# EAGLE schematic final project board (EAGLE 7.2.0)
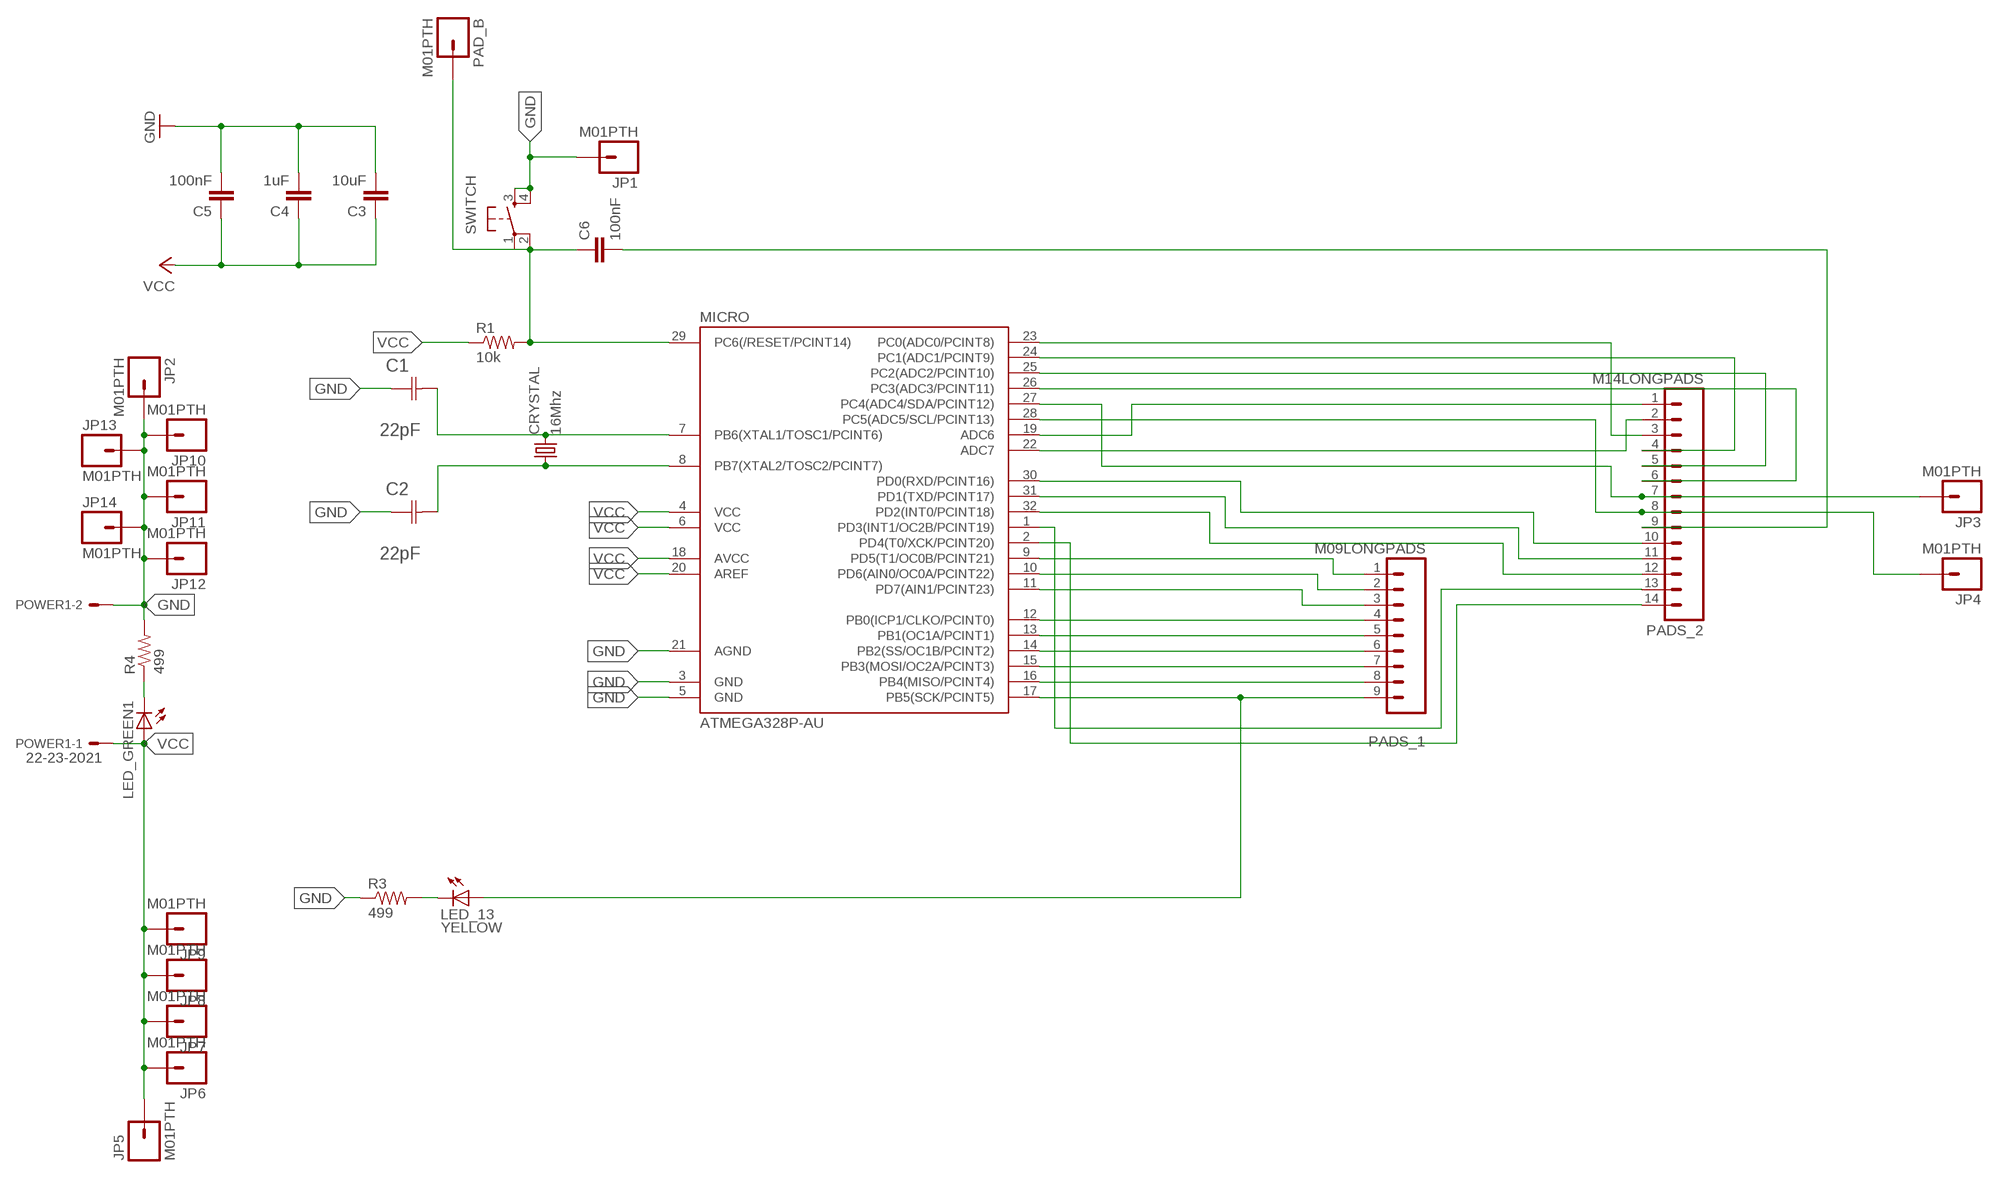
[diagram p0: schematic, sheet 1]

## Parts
C1  22pF  0612ZC225MAT2A  [CAPC3216X178N]
C2  22pF  0612ZC225MAT2A  [CAPC3216X178N]
C3  10uF  CAP1206  [1206]
C4  1uF  CAP1206  [1206]
C5  100nF  CAP1206  [1206]
C6  100nF  CAP1206  [1206]
CRYSTAL  16Mhz  CSM-7X-DU  [CSM-7X-DU]
JP1  M01PTH  [1X01]
JP2  M01PTH  [1X01]
JP3  M01PTH  [1X01]
JP4  M01PTH  [1X01]
JP5  M01PTH  [1X01]
JP6  M01PTH  [1X01]
JP7  M01PTH  [1X01]
JP8  M01PTH  [1X01]
JP9  M01PTH  [1X01]
JP10  M01PTH  [1X01]
JP11  M01PTH  [1X01]
JP12  M01PTH  [1X01]
JP13  M01PTH  [1X01]
JP14  M01PTH  [1X01]
LED_13  YELLOW  LED1206  [1206]
LED_GREEN1  LED1206  [1206]
MICRO  ATMEGA328P-AU  ATMEGA48/88/168-AU  [TQFP32-08]
PAD_B  M01PTH  [1X01]
PADS_1  M09LONGPADS  [1X09_LONGPADS]
PADS_2  M14LONGPADS  [1X14-LONGPADS]
POWER1  22-23-2021  [22-23-2021]
R1  10k  RESISTOR1206  [1206]
R3  499  RESISTOR1206  [1206]
R4  499  RESISTOR1206  [1206]
SWITCH  6MM_SWITCH6MM_SWITCH  [6MM_SWITCH]

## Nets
GND: C1.1(C1) C2.1(C1) C3.2 C4.2 C5.2 JP1.1 JP2.1 JP10.1 JP11.1 JP12.1 JP13.1 JP14.1 MICRO.3(GND) MICRO.5(GND) MICRO.21(AGND) POWER1.2 R3.1 R4.2 SWITCH.3(S) SWITCH.4(S1)
N$1: MICRO.9(PD5(T1/OC0B/PCINT21)) PADS_1.1
N$2: C1.2(C2) CRYSTAL.2 MICRO.7(PB6(XTAL1/TOSC1/PCINT6))
N$3: C6.2 PADS_2.9
N$4: MICRO.10(PD6(AIN0/OC0A/PCINT22)) PADS_1.2
N$5: MICRO.11(PD7(AIN1/PCINT23)) PADS_1.3
N$6: MICRO.12(PB0(ICP1/CLKO/PCINT0)) PADS_1.4
N$7: MICRO.13(PB1(OC1A/PCINT1)) PADS_1.5
N$8: MICRO.14(PB2(SS/OC1B/PCINT2)) PADS_1.6
N$9: C2.2(C2) CRYSTAL.1 MICRO.8(PB7(XTAL2/TOSC2/PCINT7))
N$10: MICRO.15(PB3(MOSI/OC2A/PCINT3)) PADS_1.7
N$11: MICRO.16(PB4(MISO/PCINT4)) PADS_1.8
N$12: LED_13.1(A) MICRO.17(PB5(SCK/PCINT5)) PADS_1.9
N$13: MICRO.19(ADC6) PADS_2.1
N$14: MICRO.22(ADC7) PADS_2.2
N$15: MICRO.23(PC0(ADC0/PCINT8)) PADS_2.3
N$16: MICRO.24(PC1(ADC1/PCINT9)) PADS_2.4
N$17: MICRO.25(PC2(ADC2/PCINT10)) PADS_2.5
N$18: MICRO.26(PC3(ADC3/PCINT11)) PADS_2.6
N$19: JP3.1 MICRO.27(PC4(ADC4/SDA/PCINT12)) PADS_2.7
N$20: MICRO.30(PD0(RXD/PCINT16)) PADS_2.10
N$21: MICRO.31(PD1(TXD/PCINT17)) PADS_2.11
N$22: MICRO.32(PD2(INT0/PCINT18)) PADS_2.12
N$23: MICRO.1(PD3(INT1/OC2B/PCINT19)) PADS_2.13
N$24: MICRO.2(PD4(T0/XCK/PCINT20)) PADS_2.14
N$25: JP4.1 MICRO.28(PC5(ADC5/SCL/PCINT13)) PADS_2.8
N$27: LED_13.2(C) R3.2
N$28: C6.1 MICRO.29(PC6(/RESET/PCINT14)) PAD_B.1 R1.2 SWITCH.1(P) SWITCH.2(P1)
N$29: LED_GREEN1.2(C) R4.1
VCC: C3.1 C4.1 C5.1 JP5.1 JP6.1 JP7.1 JP8.1 JP9.1 LED_GREEN1.1(A) MICRO.4(VCC) MICRO.6(VCC) MICRO.18(AVCC) MICRO.20(AREF) POWER1.1 R1.1

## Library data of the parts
C1 C2 = AVX_By_element14_Batch_1:0612ZC225MAT2A: Capacitor 1206; MPN: 0612ZC225MAT2A; OC_FARNELL: -; OC_NEWARK: 12N3209; SUPPLIER: AVX; TOLERANCE: ±20%; VALUE: 2.2µF; VOLTAGERATING: 10V
C3-C6 = 01_SparkFun:CAP: Capacitor
CRYSTAL = 01_FAB_Hello:CSM-7X-DU: SMD CRYSTAL; OC_FARNELL: unknown; OC_NEWARK: unknown
JP1-JP14 PAD_B = 01_SparkFun:M01: Header 1
LED_13 LED_GREEN1 = 01_FAB_Hello:LED
MICRO = atmega8:ATMEGA48/88/168
PADS_1 = 01_SparkFun:M09: Header 9 Standard 9-pin 0.1" header. Use with straight break away headers (SKU : PRT-00116), right angle break away headers (PRT-00553), swiss pins (PRT-00743), machine pins (PRT-00117), and female headers (PRT-00115).
PADS_2 = 01_SparkFun:M14: Header 14 Standard 14-pin 0.1" header. Use with straight break away headers (SKU : PRT-00116), right angle break away headers (PRT-00553), swiss pins (PRT-00743), machine pins (PRT-00117), and female headers (PRT-00115).
POWER1 = con-molex:22-23-2021: .100" (2.54mm) Center Header - 2 Pin; MF: MOLEX; MPN: 22-23-2021; OC_FARNELL: 1462926; OC_NEWARK: 25C3832
R1 R3 R4 = 01_SparkFun:RESISTOR: Resistor
SWITCH = 01_FAB_Hello:6MM_SWITCH: OMRON SWITCH

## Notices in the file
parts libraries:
01_SparkFun: Licensing: CC v3.0 Share-Alike You are welcome to use this library for commercial purposes.
